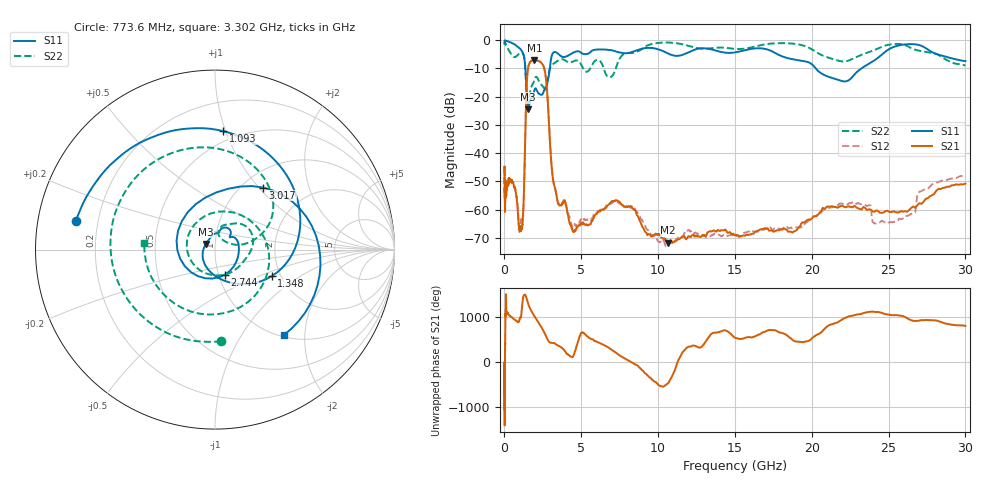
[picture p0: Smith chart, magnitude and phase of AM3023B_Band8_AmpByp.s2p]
# Hz S DB R 50.0
!freq dBS11 angS11 dBS21 angS21 dBS12 angS12 dBS22 angS22
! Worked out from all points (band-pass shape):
!   1601 points, 10 MHz to 30 GHz, reference 50 ohm
!   highest |S21| = -7.10 dB at 1.952 GHz (marker M1); lowest = -71.7 dB at 10.65 GHz (marker M2)
!   |S21| within 3 dB of the highest: 1.531 GHz to 2.59 GHz (1.059 GHz wide, 51.4 % of centre)
!   lowest |S11| = -24.5 dB at 1.551 GHz (marker M3), VSWR 1.13, Z = 45.1 + j2.9 ohm
!   |S11| at or under -10 dB: 1.359 GHz to 2.956 GHz (1.597 GHz wide, 74 % of centre); 20.25 GHz to 23.25 GHz (3.004 GHz wide, 13.8 % of centre)
!   |S22| runs from -23.2 to -0.9 dB; largest |S21 - S12| = 0.01
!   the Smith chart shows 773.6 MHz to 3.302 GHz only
!   S11 on the Smith chart (normalised r, x): 773.6 MHz: 0.12, +0.10; 1.093 GHz: 0.42, +0.98; 1.348 GHz: 1.79, -0.61; 2.744 GHz: 1.07, -0.31; 3.017 GHz: 1.23, +1.06; 3.302 GHz: 1.03, -1.57
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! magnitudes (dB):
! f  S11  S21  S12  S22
! 10 MHz  -0.4  -44.8  -44.7  -0.9
! 38.04 MHz  -0.2  -59.9  -59.6  -1.0
! 50.6 MHz  -0.4  -50.8  -52.2  -1.3
! 144.7 MHz  -0.4  -52.8  -50.4  -2.1
! 547.7 MHz  -1.3  -50.4  -50.3  -5.9
! 773.6 MHz  -2.0  -54.9  -55.1  -5.8
! 1.093 GHz  -3.6  -66.9  -64.1  -4.5
! 1.22 GHz  -4.9  -60.4  -62.6  -5.0
! 1.348 GHz  -9.2  -35.6  -36.0  -9.8
! 1.551 GHz  -24.5  -9.5  -9.5  -22.9
! 1.952 GHz  -17.7  -7.1  -7.1  -14.1
! 2.084 GHz  -17.6  -7.2  -7.2  -13.1
! 2.744 GHz  -16.5  -16.1  -16.1  -15.2
! 3.017 GHz  -7.2  -41.2  -40.8  -9.4
! 3.302 GHz  -4.3  -52.5  -52.7  -8.0
! 4.503 GHz  -4.4  -67.7  -66.1  -7.5
! 7.926 GHz  -4.7  -59.0  -58.5  -4.6
! 10.65 GHz  -4.8  -71.7  -72.4  -0.9
! 16.79 GHz  -3.0  -66.9  -67.0  -1.7
! 21.78 GHz  -14.2  -59.1  -58.0  -7.4
! 24.93 GHz  -3.6  -60.4  -64.9  -1.8
! 30 GHz  -7.5  -50.8  -47.9  -9.1
